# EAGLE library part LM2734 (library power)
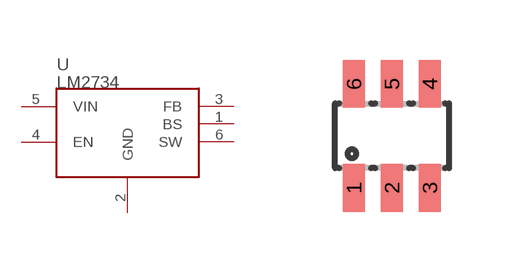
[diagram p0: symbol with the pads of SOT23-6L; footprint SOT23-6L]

Designator prefix U

## LM2734  [SOT23-6L]
1  BS
2  GND
3  FB
4  EN
5  VIN
6  SW

## Footprint SOT23-6L (pad centres in mm)
Small Outline Transistor
smd 0.55 x 1.2: 1 -0.95,-1.3; 2 0,-1.3; 3 0.95,-1.3; 4 0.95,1.3; 5 0,1.3; 6 -0.95,1.3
